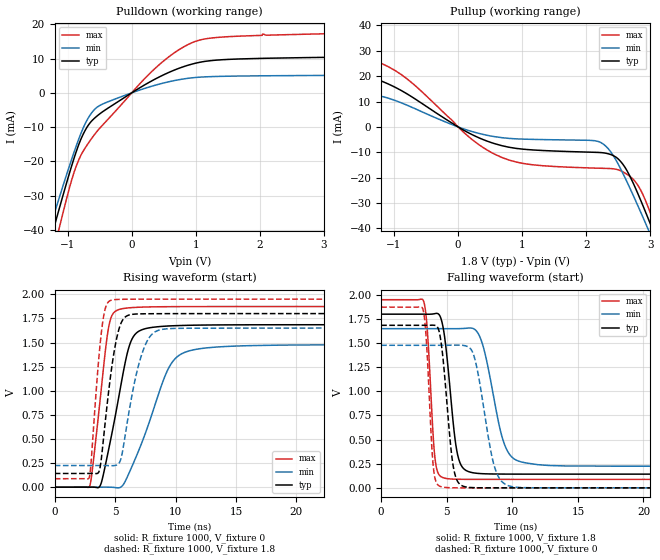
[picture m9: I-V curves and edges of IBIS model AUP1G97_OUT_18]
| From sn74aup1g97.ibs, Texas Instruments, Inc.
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[Model]   AUP1G97_OUT_18
Model_type  Output
Vref =   0
Rref =   1E6
Cref =   30p
Vmeas =   0.9
| variable   typ   min   max
C_comp   2.80pF   1.94pF   4.08pF
| C_pullup   3.08pF   1.94pF   4.08pF
| C_pulldown   2.52pF   2.14pF   3.04pF
[Temperature Range]   40   100   -40
| Ambient temperature   25   85   -40
[Voltage range]   1.8   1.65   1.95
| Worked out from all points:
|   slope of the pulldown table from 0 to 0.27 V, typ, clamps not added: 88.6 ohm
|   slope of the pullup table from 0 to 0.27 V, typ, clamps not added: 73.6 ohm
|   rising waveform, R_fixture 1000, V_fixture 0: 20-80 % time 1.55ns typ, 2.56ns min, 980ps max; typ from 0 V to 1.68 V
|   falling waveform, R_fixture 1000, V_fixture 1.8: 20-80 % time 739ps typ, 1.29ns min, 457ps max; typ from 1.8 V to 0.142 V
|   rising waveform, R_fixture 1000, V_fixture 1.8: 20-80 % time 996ps typ, 1.38ns min, 711ps max; typ from 0.142 V to 1.8 V
|   falling waveform, R_fixture 1000, V_fixture 0: 20-80 % time 670ps typ, 1.1ns min, 425ps max; typ from 1.68 V to 0 V
[Pulldown]
| AUP1G97_OUT_18
|   Voltage   I(typ)   I(min)   I(max)
-3.6V     -208.6mA   -189.9mA   -231.7mA
-1.27V    -43.16mA   -39.01mA   -50.14mA
-1.215V   -39.42mA   -35.66mA   -45.88mA
-1.125V   -33.38mA   -30.25mA   -38.97mA
-850mV    -16.31mA   -14.68mA   -20.63mA
-710mV    -10.41mA   -8.408mA   -15.6mA
-555mV    -6.973mA   -4.411mA   -11.55mA
360mV     3.96mA     2.185mA    7.039mA
705mV     6.927mA    3.722mA    12.18mA
1.03V     8.784mA    4.527mA    15.22mA
2.04V     10.05mA    4.966mA    17.1mA
7.2V      11.18mA    5.355mA    18.77mA
[Pullup]
| AUP1G97_OUT_18
|   Voltage   I(typ)   I(min)   I(max)
-3.6V     32.09mA    19.71mA    43.84mA
-3.16V    27.19mA    16.62mA    37.96mA
-2.12V    17.93mA    10.78mA    26.5mA
-1.525V   19.29mA    11.78mA    27.75mA
-1.155V   17.65mA    11.82mA    24.55mA
680mV     -7.373mA   -4.228mA   -12mA
2.185V    -10.05mA   -5.721mA   -16.26mA
2.485V    -12.35mA   -14.1mA    -16.81mA
2.725V    -21.81mA   -26.61mA   -20.47mA
2.94V     -34.55mA   -38.91mA   -30.08mA
3.085V    -43.74mA   -47.5mA    -39.77mA
7.2V      -334.8mA   -315.6mA   -357.6mA
[Ramp]
| AUP1G97_OUT_18
| variable   typ   min   max
dV/dt_r   1.01/1.56E-09   0.89/2.57E-09   1.13/9.83E-10
dV/dt_f   1.00/7.44E-10   0.86/1.30E-09   1.12/4.63E-10
R_load = 1000
[Rising Waveform]
| AUP1G97_OUT_18
R_fixture =   1000
C_fixture =   0
L_fixture =   0
V_fixture =   0
V_fixture_min = 0
V_fixture_max = 0
|   Time   V(typ)   V(min)   V(max)
0s        17.12nV    87.22nV    1.127nV
2.895ns   348.8uV    -11.01uV   13.27mV
3.75ns    13.84mV    333.1uV    900.6mV
4.4ns     355mV      465.9uV    1.615V
5.195ns   864.4mV    -6.99mV    1.837V
6.02ns    1.398V     110.9mV    1.858V
6.635ns   1.583V     286.4mV    1.864V
9.31ns    1.671V     1.206V     1.872V
10.8ns    1.678V     1.4V       1.873V
35.9ns    1.685V     1.477V     1.873V
[Falling Waveform]
| AUP1G97_OUT_18
R_fixture =   1000
C_fixture =   0
L_fixture =   0
V_fixture =   1.8
V_fixture_min = 1.65
V_fixture_max = 1.95
|   Time   V(typ)   V(min)   V(max)
0s        1.8V       1.65V      1.95V
3.25ns    1.8V       1.65V      1.93V
4.095ns   1.806V     1.65V      316.7mV
4.7ns     1.678V     1.65V      106.7mV
5.755ns   393.9mV    1.65V      89.38mV
6.66ns    168.3mV    1.656V     88.16mV
7.61ns    147.7mV    1.536V     87.95mV
9.275ns   142.9mV    501mV      87.9mV
10.46ns   142.4mV    277.9mV    87.89mV
35.9ns    142.2mV    224.7mV    87.89mV
[Rising Waveform]
| AUP1G97_OUT_18
R_fixture =   1000
C_fixture =   0
L_fixture =   0
V_fixture =   1.8
V_fixture_min = 1.65
V_fixture_max = 1.95
|   Time   V(typ)   V(min)   V(max)
0s        142.2mV    224.7mV    87.89mV
2.85ns    142.4mV    224.7mV    97.75mV
3.73ns    193.1mV    224.8mV    1.453V
4.125ns   614.3mV    224.5mV    1.825V
4.595ns   1.131V     223.4mV    1.935V
5.145ns   1.556V     230.4mV    1.946V
5.68ns    1.744V     420.8mV    1.948V
7.075ns   1.797V     1.327V     1.95V
8.545ns   1.799V     1.625V     1.95V
35.9ns    1.8V       1.65V      1.95V
[Falling Waveform]
| AUP1G97_OUT_18
R_fixture =   1000
C_fixture =   0
L_fixture =   0
V_fixture =   0
V_fixture_min = 0
V_fixture_max = 0
|   Time   V(typ)   V(min)   V(max)
0s        1.685V     1.478V     1.873V
3.175ns   1.685V     1.477V     1.855V
3.97ns    1.686V     1.477V     225.8mV
4.505ns   1.563V     1.478V     15.08mV
5.465ns   249.1mV    1.479V     847uV
6.24ns    17.28mV    1.477V     107.3uV
7.065ns   2.061mV    1.371V     18.02uV
8.57ns    116.9uV    252.6mV    1.417uV
9.675ns   26.44uV    23.38mV    531.7nV
35.9ns    -33.76nV   23.67nV    -22.31nV
